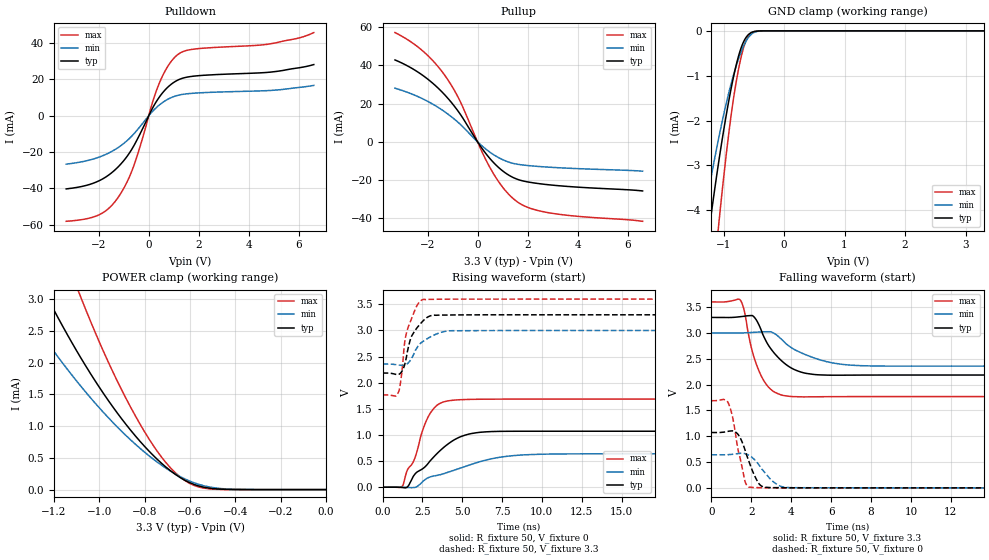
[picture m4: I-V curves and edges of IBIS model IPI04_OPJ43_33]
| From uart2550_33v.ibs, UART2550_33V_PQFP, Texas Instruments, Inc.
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[Model]   IPI04_OPJ43_33
Model_type  I/O
Vinl = 0
Vinh = 3.3
Enable   Active-Low
Vref =   1.65
Rref =   50
Cref =   15p
Vmeas =   1.65
| variable   typ   min   max
C_comp   0.75pF   0.63pF   0.84pF
| C_pullup   1.91pF   0.60pF   2.69pF
| C_pulldown   1.68pF   0.86pF   2.54pF
| C_tri-state   0.75pF   0.63pF   0.84pF
[Temperature Range]   40   125   -40
| Ambient temperature   25   110   -40
[Voltage range]   3.3   3   3.6
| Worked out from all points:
|   slope of the pulldown table from 0 to 0.495 V, typ, clamps not added: 42.5 ohm
|   slope of the pullup table from 0 to 0.495 V, typ, clamps not added: 56.6 ohm
|   GND clamp passes 1 mA (typ) near -0.83 V on its own axis
|   POWER clamp passes 1 mA (typ) near -0.88 V on its own axis
|   rising waveform, R_fixture 50, V_fixture 0: 20-80 % time 2.3ns typ, 3.8ns min, 1.3ns max; typ from 0 V to 1.07 V
|   falling waveform, R_fixture 50, V_fixture 3.3: 20-80 % time 1.2ns typ, 1.85ns min, 798ps max; typ from 3.3 V to 2.19 V
|   rising waveform, R_fixture 50, V_fixture 3.3: 20-80 % time 792ps typ, 1.11ns min, 644ps max; typ from 2.19 V to 3.3 V
|   falling waveform, R_fixture 50, V_fixture 0: 20-80 % time 620ps typ, 829ps min, 497ps max; typ from 1.07 V to 0 V
[GND Clamp]
| IPI04_OPJ43_33
|   Voltage   I(typ)   I(min)   I(max)
-3.3V     -33.05mA   -25.21mA   -45.94mA
-1.365V   -5.77mA    -4.499mA   -8.522mA
-1.335V   -5.445mA   -4.258mA   -8.049mA
-1.235V   -4.403mA   -3.486mA   -6.52mA
-1.205V   -4.104mA   -3.264mA   -6.077mA
-1.085V   -2.97mA    -2.425mA   -4.391mA
-1.07V    -2.836mA   -2.326mA   -4.191mA
-900mV    -1.466mA   -1.312mA   -2.144mA
-790mV    -760.5uA   -780.8uA   -1.136mA
-665mV    -234.9uA   -328.9uA   -360.8uA
-535mV    -34.57uA   -70.19uA   -41.17uA
3.3V      120.5pA    456.7nA    85.53pA
[POWER Clamp]
| IPI04_OPJ43_33
|   Voltage   I(typ)   I(min)   I(max)
-3.3V     27.38mA    19.89mA    38.28mA
-1.36V    3.994mA    3.019mA    5.927mA
-1.225V   3.005mA    2.305mA    4.439mA
-1.08V    2.071mA    1.626mA    3.023mA
-960mV    1.406mA    1.135mA    2.011mA
-840mV    843.7uA    713.5uA    1.159mA
-745mV    480uA      435.4uA    607.9uA
-685mV    294.2uA    290uA      339.2uA
-645mV    193.8uA    208.3uA    202.6uA
-585mV    85.41uA    111.8uA    69.83uA
-510mV    20.42uA    38.26uA    9.817uA
-47.99fV  120.5pA    479.3pA    97.92pA
[Pulldown]
| IPI04_OPJ43_33
|   Voltage   I(typ)   I(min)   I(max)
-3.3V     -40.27mA   -26.63mA   -58.11mA
-1.985V   -35.79mA   -22.77mA   -54.53mA
-1.565V   -32.27mA   -20.25mA   -50.55mA
-1.19V    -27.67mA   -17.18mA   -44.28mA
-600mV    -16.61mA   -10.03mA   -27.64mA
160mV     4.407mA    2.542mA    7.775mA
425mV     10.33mA    5.975mA    18.02mA
785mV     16.05mA    9.264mA    27.72mA
1.16V     19.65mA    11.24mA    33.7mA
1.865V    21.94mA    12.51mA    36.83mA
4.86V     24.05mA    13.96mA    39.63mA
6.6V      28.21mA    16.74mA    45.85mA
[Pullup]
| IPI04_OPJ43_33
|   Voltage   I(typ)   I(min)   I(max)
-3.3V     42.76mA    27.98mA    57.05mA
-2.215V   34.92mA    22.6mA     47.73mA
-1.745V   30.06mA    19.33mA    41.77mA
-1.32V    24.65mA    15.76mA    34.9mA
-715mV    14.86mA    9.436mA    21.67mA
125mV     -2.443mA   -1.519mA   -3.711mA
545mV     -9.491mA   -5.878mA   -14.58mA
1.035V    -15.51mA   -9.506mA   -24.23mA
1.535V    -19.29mA   -11.58mA   -30.82mA
2.085V    -21.14mA   -12.49mA   -34.63mA
2.95V     -22.59mA   -13.33mA   -37.29mA
6.6V      -25.67mA   -15.35mA   -41.53mA
[Ramp]
| IPI04_OPJ43_33
| variable   typ   min   max
dV/dt_r   0.65/2.33E-09   0.39/3.81E-09   1.02/1.32E-09
dV/dt_f   0.69/1.24E-09   0.40/1.89E-09   1.13/8.22E-10
R_load = 50
[Rising Waveform]
| IPI04_OPJ43_33
R_fixture =   50
C_fixture =   0
L_fixture =   0
V_fixture =   0
V_fixture_min = 0
V_fixture_max = 0
|   Time   V(typ)   V(min)   V(max)
0s        -5.807uV   -10.82uV   -1.536uV
1.25ns    -5.83mV    38.12uV    23.2mV
1.545ns   3.004mV    -3.678mV   321.8mV
2.015ns   246.2mV    -3.757mV   549.6mV
2.865ns   458.7mV    183mV      1.349V
3.38ns    633.4mV    224.6mV    1.56V
3.995ns   801.6mV    276.1mV    1.646V
5.575ns   1.028V     437.5mV    1.682V
8.8ns     1.072V     618.1mV    1.687V
24.99ns   1.072V     640.1mV    1.687V
[Falling Waveform]
| IPI04_OPJ43_33
R_fixture =   50
C_fixture =   0
L_fixture =   0
V_fixture =   3.3
V_fixture_min = 3
V_fixture_max = 3.6
|   Time   V(typ)   V(min)   V(max)
0s        3.3V       3V         3.6V
1.455ns   3.315V     2.999V     3.632V
1.65ns    3.324V     3.002V     3.422V
2.055ns   3.336V     3.01V      2.636V
2.44ns    3.106V     3.019V     2.215V
2.965ns   2.7V       3.023V     1.912V
3.625ns   2.424V     2.836V     1.787V
4.765ns   2.216V     2.572V     1.762V
7.205ns   2.183V     2.371V     1.767V
24.99ns   2.185V     2.357V     1.767V
[Rising Waveform]
| IPI04_OPJ43_33
R_fixture =   50
C_fixture =   0
L_fixture =   0
V_fixture =   3.3
V_fixture_min = 3
V_fixture_max = 3.6
|   Time   V(typ)   V(min)   V(max)
0s        2.185V     2.357V     1.767V
815ps     2.161V     2.347V     1.744V
1.025ns   2.163V     2.338V     1.841V
1.16ns    2.197V     2.335V     2.081V
1.29ns    2.263V     2.334V     2.468V
1.49ns    2.485V     2.352V     2.943V
1.82ns    2.889V     2.467V     3.229V
2.54ns    3.184V     2.792V     3.593V
4.34ns    3.297V     2.996V     3.6V
24.99ns   3.3V       3V         3.6V
[Falling Waveform]
| IPI04_OPJ43_33
R_fixture =   50
C_fixture =   0
L_fixture =   0
V_fixture =   0
V_fixture_min = 0
V_fixture_max = 0
|   Time   V(typ)   V(min)   V(max)
0s        1.071V     639.9mV    1.687V
865ps     1.097V     643.5mV    1.625V
1.07ns    1.103V     650.4mV    1.353V
1.375ns   1.013V     665.3mV    666.5mV
1.675ns   744.9mV    663.5mV    139.1mV
1.885ns   506mV      631.6mV    12.45mV
2.505ns   36.08mV    377.1mV    3.947mV
3.195ns   3.95mV     90.4mV     968.9uV
3.845ns   2.221mV    6.316mV    265.6uV
24.99ns   1.797uV    1.208uV    582.4nV
